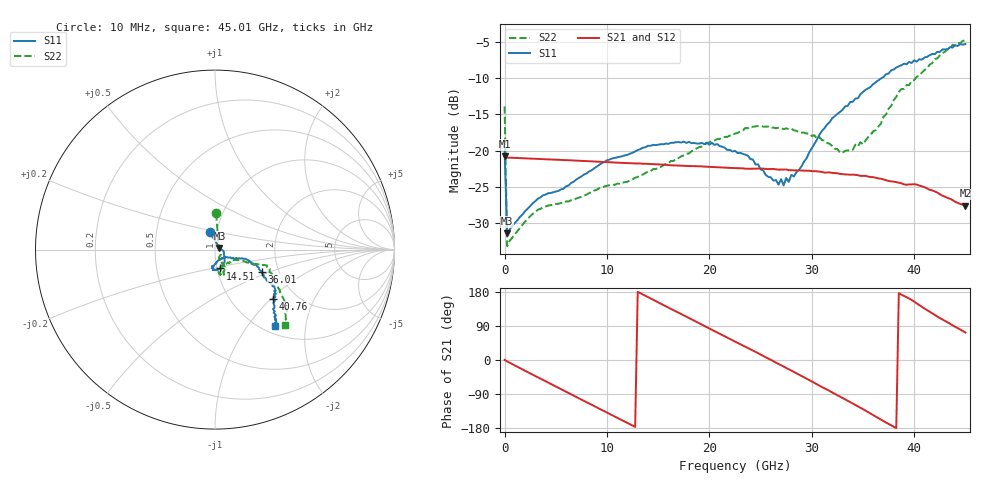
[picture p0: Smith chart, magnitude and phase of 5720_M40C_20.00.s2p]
! Device:  ADRF5720
! Description: 0.5dB LSB GaAs MMIC 6-bit Digital Attenuator
! Frequency:  0.000009 -  40 GHz
! Ports:
!	RF1	= Port 1
!	RF2	= Port 2
! Vdd:  3.3 Volt
! Vss:  -3.3 Volt
! Control:  0/3.3 Volt
! State:  20.00 dB attenuation
! Data:  The device was measured using G-S-G Probes on a matrix board.
!  Data was collected using an calibrated 4 port network analyzer.
!  The reference plane for this measurement is at the launchers.
! Note:  Analog Devices supplies this data as a sample of measured data
!  for this product.  Your particular data for this product may vary.
!  Data was taken at -40 degrees C.
!  Analog Devices reserves the right to change this data at anytime.
# GHZ S DB R 45.0
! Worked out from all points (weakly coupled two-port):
!   181 points, 10 MHz to 45.01 GHz, reference 45 ohm
!   highest |S21| = -20.80 dB at 10 MHz (marker M1); lowest = -27.6 dB at 45.01 GHz (marker M2)
!   lowest |S11| = -31.4 dB at 260 MHz (marker M3), VSWR 1.05, Z = 47.3 + j0.893 ohm
!   |S11| at or under -10 dB: start of sweep to 36.83 GHz
!   |S22| runs from -33.2 to -4.8 dB; largest |S21 - S12| = 0.00032
!   S11 on the Smith chart (normalised r, x): 10 MHz: 0.93, +0.18; 14.51 GHz: 1.04, -0.22; 36.01 GHz: 1.63, -0.44; 40.76 GHz: 1.54, -1.03; 45.01 GHz: 1.13, -1.37
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0.01  -19.98 106.7  -20.80 0.3  -20.82 0.3  -13.92 88.1
0.26  -31.45 20.6  -20.98 -3.8  -21.00 -3.9  -33.21 21.7
3.26  -26.65 -8.8  -21.16 -45.8  -21.19 -45.9  -28.18 -29.3
7.76  -23.31 -39.3  -21.45 -107.8  -21.47 -107.9  -26.22 -62.0
14.51  -19.21 -73.9  -21.88 159.1  -21.90 159.0  -22.58 -64.2
15.26  -19.13 -77.4  -21.93 148.6  -21.95 148.5  -22.26 -63.0
20.26  -18.93 -95.4  -22.27 79.6  -22.29 79.5  -18.74 -62.0
22.76  -20.35 -100.5  -22.44 45.3  -22.46 45.2  -17.58 -68.4
24.01  -21.19 -93.2  -22.52 28.4  -22.54 28.3  -16.69 -70.2
27.26  -24.81 -60.4  -22.63 -17.3  -22.65 -17.4  -17.05 -76.6
27.51  -23.80 -53.1  -22.62 -21.0  -22.64 -21.1  -16.94 -77.9
27.76  -24.34 -50.5  -22.71 -24.6  -22.73 -24.7  -17.05 -76.9
28.76  -22.68 -35.6  -22.74 -38.7  -22.77 -38.8  -17.46 -79.7
30.26  -19.08 -24.0  -22.85 -60.2  -22.88 -60.4  -17.89 -79.1
33.01  -14.39 -17.9  -23.27 -100.1  -23.30 -100.2  -20.32 -59.0
35.01  -11.91 -22.1  -23.51 -129.7  -23.54 -129.8  -19.15 -33.8
36.01  -10.83 -25.2  -23.68 -145.4  -23.71 -145.6  -17.33 -25.9
37.76  -8.93 -31.6  -24.26 -172.2  -24.28 -172.4  -13.85 -21.0
38.76  -8.22 -31.8  -24.52 172.6  -24.55 172.4  -11.51 -19.1
40.76  -7.45 -40.4  -24.94 140.5  -24.97 140.3  -9.24 -23.0
43.76  -5.78 -48.7  -26.84 91.4  -26.86 91.2  -5.39 -41.2
45.01  -5.30 -51.8  -27.62 72.5  -27.65 72.3  -4.80 -47.2
